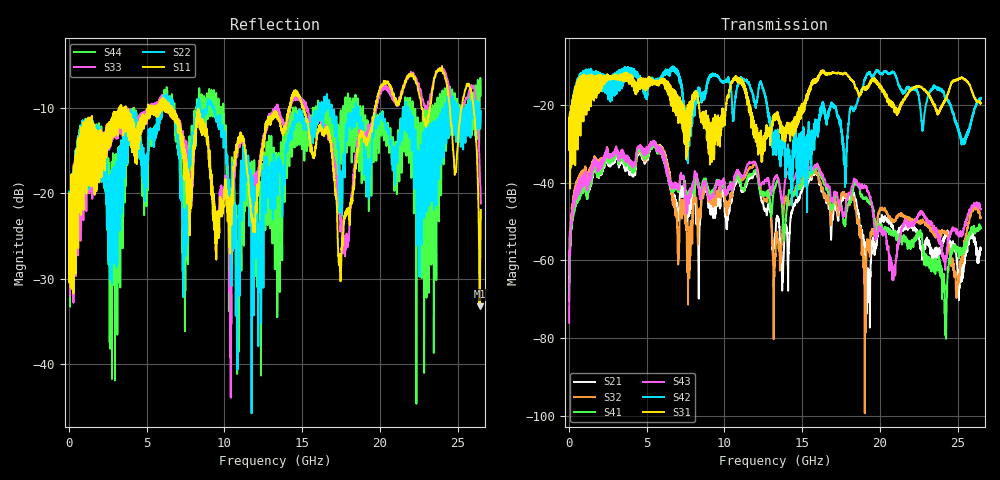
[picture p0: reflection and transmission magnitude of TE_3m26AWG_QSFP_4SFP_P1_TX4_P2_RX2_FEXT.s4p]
!Agilent Technologies,N5222A,MY51421691,A.10.00.00
!Agilent N5222A: A.10.00.00
!Date: Friday, January 30, 2015 12:37:48
!Correction: S11(Full 4 Port(1,2,3,4))
!S12(Full 4 Port(1,2,3,4))
!S13(Full 4 Port(1,2,3,4))
!S14(Full 4 Port(1,2,3,4))
!S21(Full 4 Port(1,2,3,4))
!S22(Full 4 Port(1,2,3,4))
!S23(Full 4 Port(1,2,3,4))
!S24(Full 4 Port(1,2,3,4))
!S31(Full 4 Port(1,2,3,4))
!S32(Full 4 Port(1,2,3,4))
!S33(Full 4 Port(1,2,3,4))
!S34(Full 4 Port(1,2,3,4))
!S41(Full 4 Port(1,2,3,4))
!S42(Full 4 Port(1,2,3,4))
!S43(Full 4 Port(1,2,3,4))
!S44(Full 4 Port(1,2,3,4))
!S4P File: Measurements: <S11,S12,S13,S14>,
!<S21,S22,S23,S24>,
!<S31,S32,S33,S34>,
!<S41,S42,S43,S44>:
# Hz S  dB  R 50.0
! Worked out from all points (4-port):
!   2650 points, 10 MHz to 26.5 GHz, reference 50 ohm
!   strongest paths, dB at 10 MHz, 6.63 GHz, 13.26 GHz, 19.88 GHz, 26.5 GHz:
!     S31: -24.8, -19.0, -23.3, -14.9, -19.6
!     S42: -24.7, -11.3, -30.4, -11.5, -18.3
!     S43: -76.0, -41.0, -38.8, -52.8, -46.9
!     S41: -70.4, -41.8, -41.1, -52.6, -51.7
!     S32: -63.7, -42.0, -59.7, -48.4, -49.1
!     S21: -61.7, -42.2, -53.1, -52.2, -57.3
!   lowest |S11| = -33.2 dB at 26.43 GHz (marker M1), VSWR 1.04, Z = 51.6 - j1.51 ohm
!   |S11| at or under -10 dB: start of sweep to 3.24 GHz; 6.606 GHz to 14.16 GHz (7.55 GHz wide, 72.7 % of centre); 15.11 GHz to 19.68 GHz (4.576 GHz wide, 26.3 % of centre)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
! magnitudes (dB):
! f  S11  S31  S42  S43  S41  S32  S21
! 10 MHz  -20.0  -24.8  -24.7  -76.0  -70.4  -63.7  -61.7
! 760 MHz  -12.3  -12.7  -11.9  -41.2  -42.5  -40.2  -41.9
! 5.43 GHz  -9.9  -13.9  -14.2  -30.1  -30.6  -30.3  -30.5
! 7.69 GHz  -20.4  -24.5  -27.7  -45.1  -44.1  -55.9  -48.5
! 24.19 GHz  -6.5  -19.2  -18.1  -60.4  -72.4  -52.8  -53.5
! 26.43 GHz  -33.2  -19.4  -18.4  -46.0  -51.3  -48.1  -57.7
! 26.5 GHz  -21.9  -19.6  -18.3  -46.9  -51.7  -49.1  -57.3
